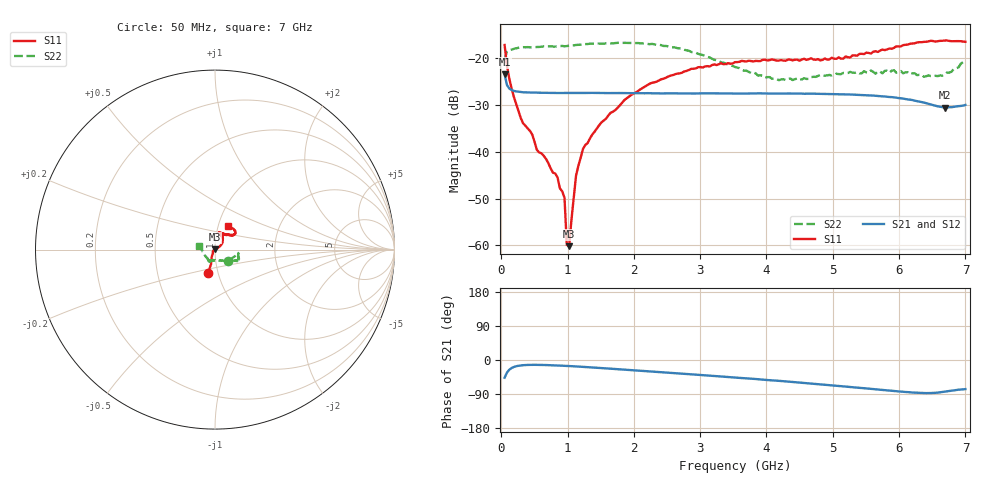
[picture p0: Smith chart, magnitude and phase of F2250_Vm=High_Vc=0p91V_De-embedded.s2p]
! Integrated Device Technology
! Corporate Headquarters
! 6024 Silver Creek Valley Road
! San Jose, CA 95138  USA
! Phone:  1-408-284-8200
! Toll Free:  1-800-223-1366
! Webpage:  http://www.idt.com/
! Timing and RF Division
! 515 Groton Road, Suite 102
! Westford, MA 01886-6024
! Device:  F2250
! Description: Voltage Variable RF Attenuator
! Frequency:  50.0 -  6000.00 MHz
! Package:  3x3 mm Thin QFN Plastic Package: 16 pin
! Ports:  2 RF, 3 DC
!  Pin  1  = GND
!  Pin  2  = NC
!  Pin  3  = RF1  = Port 1
!  Pin  4  = NC
!  Pin  5  = GND
!  Pin  6  = GND
!  Pin  7  = GND
!  Pin  8  = GND
!  Pin  9  = NC
!  Pin 10  = RF2  = Port 2
!  Pin 11  = NC
!  Pin 12  = GND
!  Pin 13  = GND
!  Pin 14  = VCNTRL
!  Pin 15  = VDD
!  Pin 16  = VMODE
! Vcntrl:  0.910 Volts
! Vmode:  +3.300 Volts
! Vdd:  +3.30  Volts
! Current:  1.313 mA
! Data:  The device was measured on a the F2250 evaluation board which has
!  individual transmission lines to the RF pins.  Data was collected
!  using a calibrated network analyzer.  The evaluation board was
!  de-embedded using a TRL calibration technique.
!  The reference plane is the edge of the package pin.
! Misc:  SN 10
!  Action Tracker AT0258
! Date Measured:  2014-11-26
! Date:  2015-10-15  MJV
! Note:
!  Integrated Device Technology supplies this data as a sample of measured
!  data at the package pin for this product.  Your particular data for this
!  product may vary.
!  Data was taken at 25 degrees C.
!  Integrated Device Technology reserves the right to change this data at anytime.
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# GHz S dB R 50
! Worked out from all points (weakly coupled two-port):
!   201 points, 50 MHz to 7 GHz, reference 50 ohm
!   highest |S21| = -23.47 dB at 50 MHz (marker M1); lowest = -30.5 dB at 6.687 GHz (marker M2)
!   lowest |S11| = -60.2 dB at 1.023 GHz (marker M3), VSWR 1.00, Z = 50.1 + j0.0799 ohm
!   |S11| at or under -10 dB: start of sweep to end of sweep
!   |S22| runs from -24.7 to -16.7 dB; largest |S21 - S12| = 0.00019
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0.05  -17.18 -106.9  -23.47 -46.7  -23.47 -46.7  -20.28 -39.1
0.1195  -24.30 -109.1  -26.45 -25.8  -26.44 -25.8  -18.28 -12.1
0.29325  -32.76 -120.8  -27.23 -14.4  -27.23 -14.4  -17.66 -9.1
0.467  -36.32 -138.2  -27.34 -12.7  -27.34 -12.7  -17.68 -9.2
0.5365  -39.59 -144.6  -27.34 -12.8  -27.36 -12.8  -17.60 -10.4
0.84925  -45.53 173.4  -27.43 -14.5  -27.42 -14.5  -17.45 -15.4
0.884  -47.80 167.8  -27.42 -14.8  -27.41 -14.8  -17.41 -16.2
0.9535  -49.83 179.2  -27.43 -15.3  -27.42 -15.4  -17.44 -16.7
0.98825  -59.88 -179.4  -27.43 -15.6  -27.43 -15.7  -17.40 -17.2
1.023  -60.17 54.5  -27.43 -15.9  -27.42 -16.0  -17.30 -17.4
1.12725  -45.11 29.3  -27.42 -16.9  -27.42 -16.9  -17.16 -18.7
1.2315  -39.43 26.2  -27.42 -18.0  -27.43 -18.1  -17.01 -20.4
1.5095  -33.73 33.0  -27.43 -21.3  -27.44 -21.4  -16.90 -22.4
1.857  -28.93 34.8  -27.45 -25.4  -27.44 -25.5  -16.71 -24.9
2.37825  -24.74 43.8  -27.51 -31.7  -27.51 -31.8  -17.12 -27.5
2.86475  -22.27 55.3  -27.53 -37.8  -27.53 -37.8  -18.65 -31.3
3.525  -20.84 70.4  -27.54 -46.3  -27.54 -46.3  -21.87 -50.4
4.18525  -20.49 76.5  -27.55 -55.0  -27.54 -55.0  -24.69 -82.6
4.7065  -20.28 71.2  -27.58 -62.7  -27.58 -62.7  -23.97 -105.0
5.85325  -17.92 39.8  -28.29 -80.7  -28.27 -80.8  -23.10 -115.5
6.68725  -16.21 47.2  -30.55 -83.6  -30.53 -83.7  -23.53 -168.8
7  -16.48 61.9  -29.98 -76.8  -29.97 -77.0  -20.58 167.3
